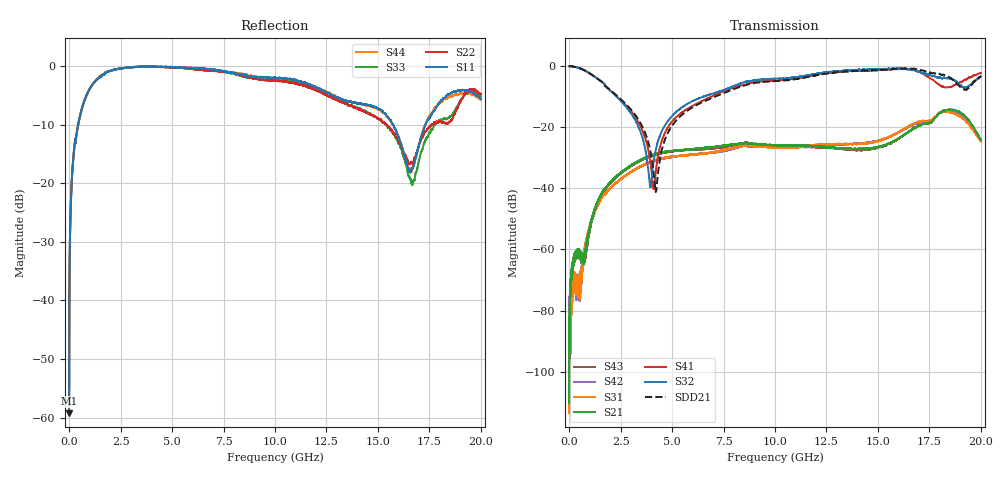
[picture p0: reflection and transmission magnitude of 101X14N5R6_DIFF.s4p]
!{101X14N5R6}
!Johanson Technology Inc.
!www.johansontechnology.com
!Test Board Conditions:
!Substrate Type  RO4350B
!Substrate Thickness  10 mil
!Substrate Dk  3.66
!TL Type: GCPW
!TL Trace Width  20 mil
!TL Gap  15 mil
!PART MODE DIFFERENTIAL
!DUT TOPOLOGY	DIFFERENTIAL 4-PORT
!Mounting Pad LxW  20x35 mil
# MHz S  dB  R 50
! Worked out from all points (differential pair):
!   20001 points, 300 kHz to 20 GHz, reference 50 ohm
!   strongest paths, dB at 300 kHz, 5 GHz, 10 GHz, 15 GHz, 20 GHz:
!     S32: 0.0, -16.3, -4.1, -1.1, -3.3
!     S41: 0.0, -18.1, -4.7, -1.3, -2.2
!     S21: -84.3, -27.7, -25.8, -26.5, -24.2
!     S31: -84.0, -29.6, -26.7, -24.6, -24.6
!     S42: -75.4, -29.8, -26.6, -24.4, -24.2
!     S43: -87.5, -27.9, -26.3, -26.7, -24.6
!   taken as a pair (ports 2,1 in; 3,4 out), SDD21 dB: 0.0, -19.5, -4.9, -1.3, -3.3
!   lowest |S11| = -59.3 dB at 1.3 MHz (marker M1), VSWR 1.00, Z = 50 - j0.108 ohm
!   |S11| at or under -10 dB: start of sweep to 433.2 MHz; 15.72465 GHz to 15.72569 GHz (1.042 MHz wide, 0.00662 % of centre); 15.73 GHz to 17.31 GHz (1.581 GHz wide, 9.57 % of centre)
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0.3  -59.21 -89.0  -79.20 -132.6  -82.31 87.7  -0.02 -0.0
     -84.34 -114.3  -58.94 -68.5  -0.01 0.0  -103.06 104.9
     -84.00 115.8  -0.03 -0.0  -51.51 -58.6  -93.08 -47.1
     -0.00 0.1  -75.42 -113.4  -87.46 52.6  -56.35 -96.3
1.3  -59.27 -82.8  -86.96 0.5  -81.49 -110.4  0.00 -0.0
     -85.42 7.5  -55.73 -32.7  -0.02 -0.0  -89.62 125.8
     -91.02 158.9  -0.02 -0.0  -55.16 -34.4  -90.73 -36.2
     -0.01 -0.0  -89.25 -153.1  -82.95 -23.1  -57.07 -87.2
318.295  -12.54 -105.8  -60.81 71.7  -70.69 43.7  -0.26 -16.0
         -62.16 72.5  -12.83 -106.4  -0.28 -16.3  -72.44 34.4
         -72.14 17.1  -0.28 -16.3  -12.74 -106.3  -62.79 67.0
         -0.27 -16.0  -70.15 15.9  -62.39 77.9  -12.56 -107.3
1829.273  -1.02 -163.3  -39.32 124.6  -41.16 139.4  -6.92 -72.2
          -39.39 124.3  -1.07 -162.1  -7.02 -71.7  -41.24 140.2
          -41.24 139.1  -7.03 -71.8  -1.03 -163.2  -39.60 124.7
          -6.92 -72.4  -41.33 139.2  -39.65 124.5  -1.06 -163.1
4106.238  -0.10 164.5  -28.91 69.9  -30.93 69.1  -40.30 -17.1
          -28.92 70.0  -0.16 160.1  -31.24 46.2  -31.14 67.8
          -30.92 68.8  -31.21 45.9  -0.13 158.7  -29.18 67.6
          -40.17 -17.6  -31.12 67.4  -29.23 67.5  -0.13 160.8
7841.182  -1.08 122.0  -25.67 6.5  -26.97 -6.7  -7.30 26.4
          -25.74 6.7  -1.09 115.6  -7.03 21.2  -27.26 -9.9
          -26.93 -6.8  -6.96 21.1  -1.23 111.8  -25.98 0.9
          -7.32 26.3  -27.27 -10.0  -26.00 1.1  -1.02 115.1
20000  -5.59 32.1  -24.23 -85.8  -24.72 -110.1  -2.26 -70.1
       -24.21 -86.1  -4.82 45.5  -3.30 -64.9  -24.22 -104.1
       -24.62 -109.5  -3.27 -64.1  -5.14 37.1  -24.56 -89.7
       -2.23 -69.9  -24.24 -103.7  -24.59 -89.8  -5.67 25.7
